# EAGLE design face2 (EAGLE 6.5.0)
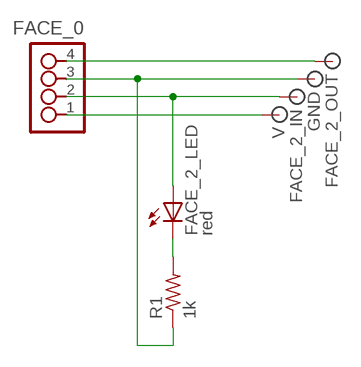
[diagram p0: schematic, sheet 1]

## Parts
FACE_0  4_PIN_HEADER  [SMT_PINS_4]
FACE_2_IN  SIGNAL  [PAD.2]
FACE_2_LED  red  LED1206  [1206]
FACE_2_OUT  SIGNAL  [PAD.2]
GND  SIGNAL  [PAD.2]
R1  1k  RESISTOR1206  [1206]
V  SIGNAL  [PAD.2]

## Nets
N$1: FACE_0.1 V.P$1
N$2: FACE_0.2 FACE_2_IN.P$1 FACE_2_LED.1(A)
N$3: FACE_0.3 GND.P$1 R1.1
N$4: FACE_0.4 FACE_2_OUT.P$1
N$5: FACE_2_LED.2(C) R1.2

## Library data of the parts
FACE_0 = ot:4_PIN_HEADER
FACE_2_IN FACE_2_OUT GND V = ot:SIGNAL: Signal
FACE_2_LED = 01_FAB_Hello:LED
R1 = 01_FAB_Hello:RESISTOR

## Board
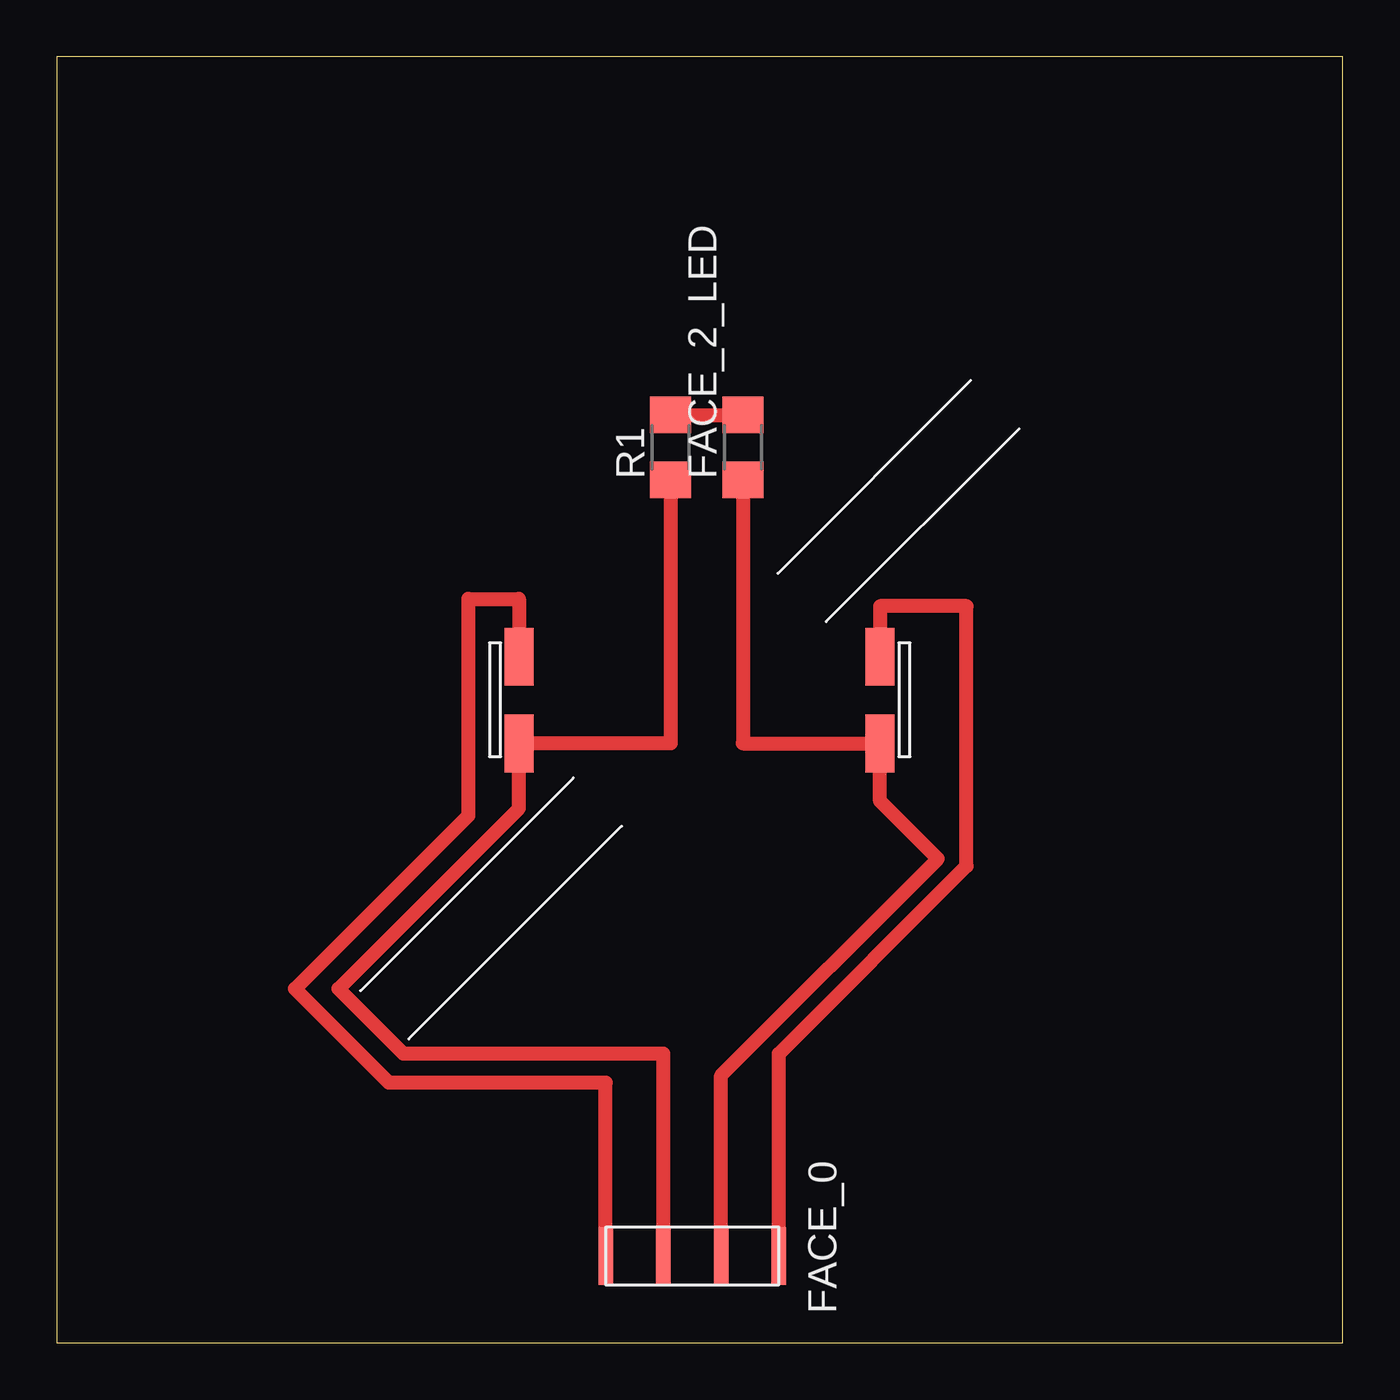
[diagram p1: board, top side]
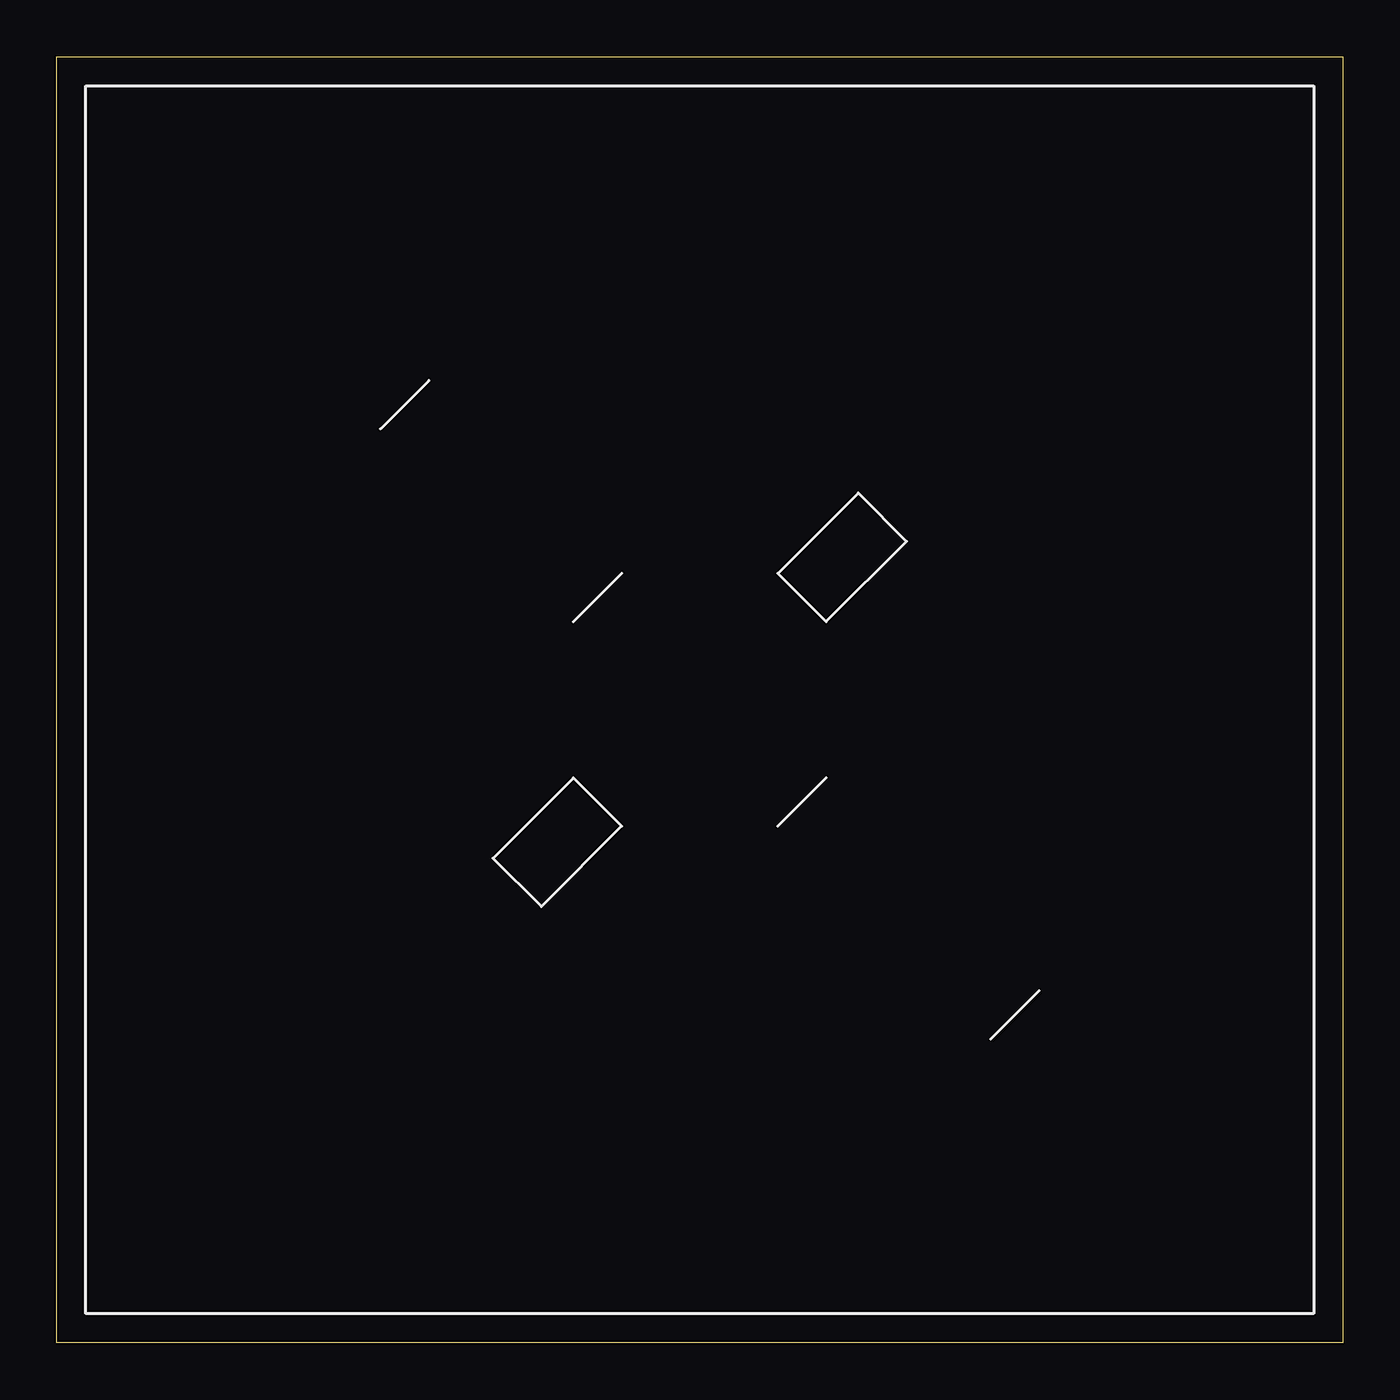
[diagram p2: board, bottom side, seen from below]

Size 56.54 x 56.54 mm. Coordinates in mm from the lower left corner, seen from the top.
Outline: 0,0 56.54,0 56.54,56.54 0,56.54 0,0
Copper layers (1*16): Top 0.035mm / dielectric 1.5mm / Bottom 0.035mm
Design rules "default *": minimum track width 10mil, minimum drill 24mil, track to track 0.4mm, track to pad 0.4mm, pad to pad 0.4mm, via to via 0.4mm, smd to smd 0.4mm, copper to edge 40mil, drill to drill 8mil, minimum pad ring 10mil, minimum via ring 8mil, stop-mask expansion 4mil, vias tented up to drill 0mil, thermal gap 10mil

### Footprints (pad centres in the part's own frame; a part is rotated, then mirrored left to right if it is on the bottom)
SMT_PINS_4 = smd 2.54 x 0.635: 1 0,0; 2 0,2.54; 3 0,5.08; 4 0,7.62
PAD.2 = smd 2.54 x 1.27: P$1 0,0
1206 = smd 1.6 x 1.803: 1 -1.422,0; 2 1.422,0

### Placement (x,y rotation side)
FACE_0  31.75,3.81 90 top
FACE_2_IN  36.2,26.35 90 top
FACE_2_LED  30.16,39.37 90 top
FACE_2_OUT  20.32,30.16 90 top
GND  20.32,26.35 90 top
R1  26.99,39.37 90 top
U$1  [CUBE_POS]  55.27,1.27 90 top
V  36.2,30.16 90 top

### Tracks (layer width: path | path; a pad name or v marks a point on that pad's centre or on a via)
N$1
  Top 0.61: FACE_0.1 31.75,12.7 40.01,20.95 40.01,32.38 36.2,32.38 V.P$1
N$2
  Top 0.61: FACE_0.2 29.21,11.75 38.73,21.27 36.2,23.81 FACE_2_IN.P$1 30.16,26.35 FACE_2_LED.1
N$3
  Top 0.61: FACE_0.3 26.67,12.7 15.24,12.7 12.38,15.56 20.32,23.5 GND.P$1 26.99,26.35 R1.1
N$4
  Top 0.61: FACE_0.4 24.13,11.43 14.61,11.43 10.48,15.56 18.1,23.18 18.1,32.7 20.32,32.7 FACE_2_OUT.P$1
N$5
  Top 0.61: R1.2 FACE_2_LED.2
